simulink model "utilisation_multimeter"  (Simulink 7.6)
settings: Solver=ode23tb  SolverMode=SingleTasking  StartTime=0.0  StopTime=0.05  RelTol=1e-4
StopFcn:
  | close all
  | load signaux_multimeter.mat
  | plot(x(1,:),x(2,:))
  | hold on
  | plot(x(1,:),x(3,:))
  | %axis([0 0.04 -20 1020])
  | grid
  | title('Tension aux bornes de C et signal de la source de tension')
  | xlabel('temps')
libraries: powerlib x11

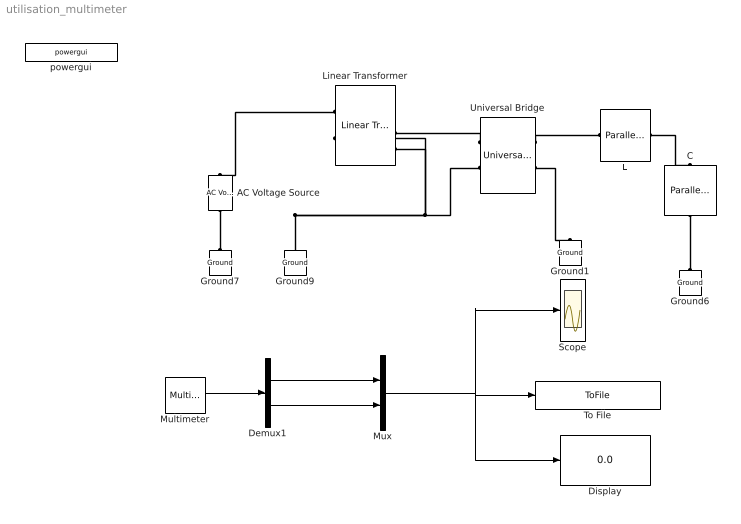
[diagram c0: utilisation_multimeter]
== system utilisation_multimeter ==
  AC Voltage Source : powerlib/Electrical Sources/AC Voltage Source  DialogController=POWERSYS.PowerSysDialog  SystemSampleTime=-1  Amplitude=220  Phase=0  Frequency=60  SampleTime=0  Measurements=Voltage
  C : powerlib/Elements/Parallel RLC Branch  DialogController=POWERSYS.PowerSysDialog  PhysicalDomain=powersysdomain  SubClassName=unknown  LeftPortType=p1  RightPortType=p1  LConnTagsString=a  RConnTagsString=__new0  BranchType=C  Resistance=1e3  Inductance=1  SetiL0=off  InitialCurrent=0  Capacitance=1e-06  Setx0=off  InitialVoltage=0  Measurements=Branch voltage
  Demux1 : Demux  Outputs=2
  Display : Display
  Ground{1,6..7,9} (4 alike) : powerlib/Elements/Ground  DialogController=POWERSYS.PowerSysDialog  PhysicalDomain=powersysdomain  SubClassName=unknown  LeftPortType=p1  RightPortType=p1  LConnTagsString=a
  L : powerlib/Elements/Parallel RLC Branch  DialogController=POWERSYS.PowerSysDialog  PhysicalDomain=powersysdomain  SubClassName=unknown  LeftPortType=p1  RightPortType=p1  LConnTagsString=a  RConnTagsString=__new0  BranchType=L  Resistance=200  Inductance=1  SetiL0=off  InitialCurrent=0  Capacitance=1e-06  Setx0=off  InitialVoltage=0  Measurements=Branch current
  Linear Transformer : powerlib/Elements/Linear Transformer  DialogController=POWERSYS.PowerSysDialog  PhysicalDomain=powersysdomain  SubClassName=unknown  LeftPortType=p1  RightPortType=p1  LConnTagsString=a|b  RConnTagsString=A|B|C|D  UNITS=SI  NominalPower=[250e6 60 ]  winding1=[7.35e+005 4.3218 0.45856]  winding2=[3.15e+005 0.7938 0.084225]  ThreeWindings=on  winding3=[3.15e+005 0.7938 0.084225]  RmLm=[1.0805e+006 2866]  Measurements=None  DataType=on
  Multimeter : powerlib/Measurements/Multimeter  Tag=PoWeRsYsTeMmEaSuReMeNt  SystemSampleTime=-1  PhasorSimulation=off  OutputType=Magnitude  sel=[2 1]  L=3  Gain=[1 1]  yselected={'Usrc: AC Voltage Source','Ub: C'};  PSBOutputType=1  PSBequivalent=0  AxesSetting=[0,0.1,-100,100]  Display=0  SavedBlockNames={}
  Mux : Mux  Inputs=2
  Scope : Scope
  To File : ToFile  Filename=signaux_multimeter.mat  MatrixName=x
  Universal Bridge : powerlib/Power Electronics/Universal Bridge  DialogController=POWERSYS.PowerSysDialog  SystemSampleTime=-1  Arms=2  SnubberResistance=1e5  SnubberCapacitance=inf  Device=Diodes  Ron=1e-3  Lon=0  ForwardVoltages="[  0  0  ]"  ForwardVoltage=0  GTOparameters=[ 10e-6 , 20e-6 ]  IGBTparameters=[ 1e-6 , 2e-6 ]  Measurements=None  Measurements_2=None  converterType=Rectifier
  powergui : powerlib/powergui  Priority=2  SystemSampleTime=-1  SimulationMode=Continuous  SampleTime=0  frequency=60  SPID=off  DisableSnubberDevices=off  DisableRonSwitches=off  DisableVfSwitches=off  SwTol=0  Interpol=off  frequencyindice=60  echomessages=off  HookPort=off  DisplayEquations=off  FunctionMessages=off  EnableUseOfTLC=off  x0status=blocks  RestoreLinks=warning  ResistiveCurrentMeasurement=off  Frange=0:1000  Ylog=off  Xlog=on  ShowGrid=on  save=off  variable=ZData  ZoomFFT=on  StartTime=0.0  cycles=2  DisplayStyle=off  fundamental=60  FreqAxis=off  MaxFrequency=1000  frequencyindicesteady=1  RmsSteady=1  display=off  Ts=0  methode=off
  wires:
  Multimeter/1 -> Demux1/1
  Demux1/1 -> Mux/1
  Demux1/2 -> Mux/2
  Mux/1 -> To File/1, Display/1, Scope/1
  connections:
  Ground6/LConn1 -- C/RConn1
  Ground7/LConn1 -- AC Voltage Source/LConn1
  L/RConn1 -- C/LConn1
  Universal Bridge/RConn1 -- L/LConn1
  Linear Transformer/LConn1 -- AC Voltage Source/RConn1
  Ground9/LConn1 -- Linear Transformer/LConn2 -- Linear Transformer/RConn4 -- Universal Bridge/LConn2
  Universal Bridge/LConn1 -- Linear Transformer/RConn3
  Universal Bridge/RConn2 -- Ground1/LConn1
